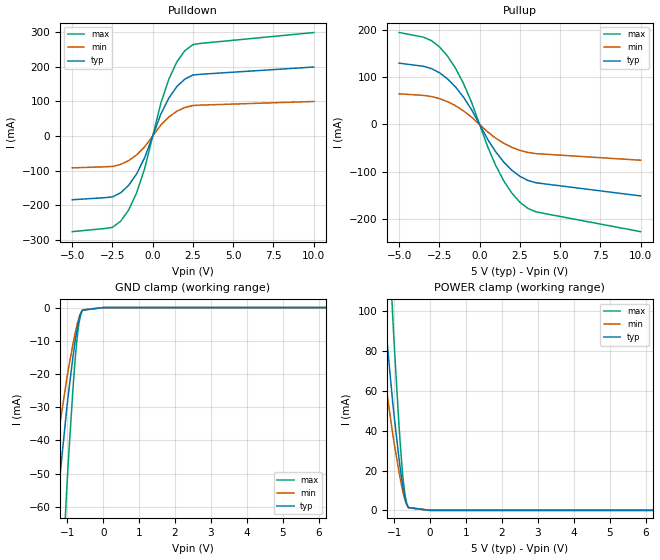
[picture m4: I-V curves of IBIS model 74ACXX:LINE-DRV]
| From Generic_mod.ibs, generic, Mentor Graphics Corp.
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[Model]   74ACXX:LINE-DRV
Model_type   I/O
Polarity   Non-Inverting
Vinl  =   0.800V
Vinh  =   2.000V
Vmeas =   1.500V
Cref  =  50.000pF
Rref  =   1.000kOhm
Vref  =   0.000V
|   typ   min   max
C_comp   10.000pF   5.000pF   15.000pF
[Voltage Range]   5.000V   4.500V   5.500V
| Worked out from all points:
|   slope of the pulldown table from 0 to 0.75 V, typ, clamps not added: 8.73 ohm
|   slope of the pullup table from 0 to 0.75 V, typ, clamps not added: 16.9 ohm
|   GND clamp passes 1 mA (typ) near -0.59 V on its own axis
[Pulldown]
| Voltage   I(typ)   I(min)   I(max)
-5V       -184mA     -91.98mA   -275.9mA
-2.5V     -175.8mA   -87.88mA   -263.6mA
-2V       -164.2mA   -82.09mA   -246.3mA
-1.5V     -142.6mA   -71.3mA    -213.9mA
-1V       -109.3mA   -54.66mA   -164mA
-500mV    -62.5mA    -31.25mA   -93.75mA
500mV     62.5mA     31.25mA    93.75mA
1V        109.3mA    54.66mA    164mA
1.5V      142.6mA    71.3mA     213.9mA
2V        164.2mA    82.09mA    246.3mA
3V        178mA      89.01mA    267mA
10V       198.8mA    99.42mA    298.3mA
[Pullup]
| Voltage   I(typ)   I(min)   I(max)
-5V       129.2mA    64.59mA    193.8mA
-3V       117.9mA    58.96mA    176.9mA
-2V       96.33mA    48.17mA    144.5mA
-1.5V     79.19mA    39.59mA    118.8mA
-1V       57.57mA    28.78mA    86.35mA
-500mV    31.25mA    15.62mA    46.88mA
500mV     -31.25mA   -15.62mA   -46.88mA
1V        -57.57mA   -28.78mA   -86.35mA
1.5V      -79.19mA   -39.59mA   -118.8mA
2.5V      -109.2mA   -54.59mA   -163.8mA
3.5V      -122.7mA   -61.37mA   -184.1mA
10V       -150.5mA   -75.26mA   -225.8mA
[GND Clamp]
| Voltage   I(typ)   I(min)   I(max)
-5V       -458.6mA   -307.2mA   -910mA
-1.008V   -29.6mA    -20.95mA   -53.03mA
-956.2mV  -24.75mA   -17.69mA   -43.53mA
-846.8mV  -15.18mA   -11.19mA   -25.05mA
-794.5mV  -11.05mA   -8.352mA   -17.33mA
-747.3mV  -7.706mA   -6.013mA   -11.33mA
-707.6mV  -5.291mA   -4.277mA   -7.25mA
-650.8mV  -2.646mA   -2.283mA   -3.218mA
-625.9mV  -1.829mA   -1.629mA   -2.116mA
-573.6mV  -748.1uA   -705.5uA   -799uA
0V        0A         0A         0A
10V       0A         0A         0A
[POWER Clamp]
| Voltage   I(typ)   I(min)   I(max)
-5V       820mA      549.2mA    1.627A
-1.036V   53.26mA    37.7mA     95.41mA
-984.1mV  44.54mA    31.82mA    78.32mA
-874.8mV  27.32mA    20.14mA    45.09mA
-822.5mV  19.88mA    15.03mA    31.19mA
-775.2mV  13.87mA    10.82mA    20.4mA
-735.6mV  9.524mA    7.699mA    13.05mA
-678.8mV  4.762mA    4.11mA     5.792mA
-653.9mV  3.293mA    2.932mA    3.809mA
-601.6mV  1.347mA    1.27mA     1.438mA
0V        0A         0A         0A
10V       0A         0A         0A
[Ramp]
|   typ   min   max
dV/dt_r   2.187V/1.800ns   1.466V/3.240ns   2.674V/1.320ns
dV/dt_f   2.555V/1.980ns   1.927V/3.564ns   2.977V/1.452ns
R_load =  50.000Ohm
|------------------- End of 74ACXX:LINE-DRV -----------------------------------
